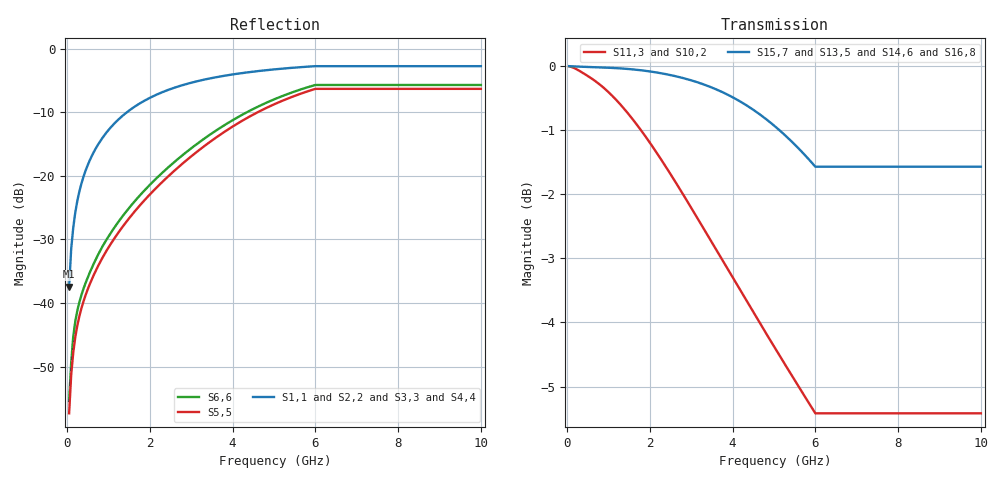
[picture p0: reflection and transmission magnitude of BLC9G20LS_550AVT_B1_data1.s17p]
! Created Mon Aug  3 12:37:55 2015
! 17 Port Network Data from SP1.SP block
! freq  magS1_1  angS1_1  magS1_2  angS1_2  magS1_3  angS1_3  magS1_4  angS1_4
!  magS1_5  angS1_5  magS1_6  angS1_6  magS1_7  angS1_7  magS1_8  angS1_8
!  magS1_9  angS1_9  magS1_10  angS1_10  magS1_11  angS1_11  magS1_12  angS1_12
!  magS1_13  angS1_13  magS1_14  angS1_14  magS1_15  angS1_15  magS1_16  angS1_16
!  magS1_17  angS1_17
!  magS2_1  angS2_1  magS2_2  angS2_2  magS2_3  angS2_3
!  magS2_4  angS2_4  magS2_5  angS2_5  magS2_6  angS2_6  magS2_7  angS2_7
!  magS2_8  angS2_8  magS2_9  angS2_9  magS2_10  angS2_10  magS2_11  angS2_11
!  magS2_12  angS2_12  magS2_13  angS2_13  magS2_14  angS2_14  magS2_15  angS2_15
!  magS2_16  angS2_16  magS2_17  angS2_17
!  magS3_1  angS3_1  magS3_2  angS3_2
!  magS3_3  angS3_3  magS3_4  angS3_4  magS3_5  angS3_5  magS3_6  angS3_6
!  magS3_7  angS3_7  magS3_8  angS3_8  magS3_9  angS3_9  magS3_10  angS3_10
!  magS3_11  angS3_11  magS3_12  angS3_12  magS3_13  angS3_13  magS3_14  angS3_14
!  magS3_15  angS3_15  magS3_16  angS3_16  magS3_17  angS3_17
!  magS4_1  angS4_1
!  magS4_2  angS4_2  magS4_3  angS4_3  magS4_4  angS4_4  magS4_5  angS4_5
!  magS4_6  angS4_6  magS4_7  angS4_7  magS4_8  angS4_8  magS4_9  angS4_9
!  magS4_10  angS4_10  magS4_11  angS4_11  magS4_12  angS4_12  magS4_13  angS4_13
!  magS4_14  angS4_14  magS4_15  angS4_15  magS4_16  angS4_16  magS4_17  angS4_17
!  magS5_1  angS5_1  magS5_2  angS5_2  magS5_3  angS5_3  magS5_4  angS5_4
!  magS5_5  angS5_5  magS5_6  angS5_6  magS5_7  angS5_7  magS5_8  angS5_8
!  magS5_9  angS5_9  magS5_10  angS5_10  magS5_11  angS5_11  magS5_12  angS5_12
!  magS5_13  angS5_13  magS5_14  angS5_14  magS5_15  angS5_15  magS5_16  angS5_16
!  magS5_17  angS5_17
!  magS6_1  angS6_1  magS6_2  angS6_2  magS6_3  angS6_3
!  magS6_4  angS6_4  magS6_5  angS6_5  magS6_6  angS6_6  magS6_7  angS6_7
!  magS6_8  angS6_8  magS6_9  angS6_9  magS6_10  angS6_10  magS6_11  angS6_11
!  magS6_12  angS6_12  magS6_13  angS6_13  magS6_14  angS6_14  magS6_15  angS6_15
!  magS6_16  angS6_16  magS6_17  angS6_17
!  magS7_1  angS7_1  magS7_2  angS7_2
!  magS7_3  angS7_3  magS7_4  angS7_4  magS7_5  angS7_5  magS7_6  angS7_6
!  magS7_7  angS7_7  magS7_8  angS7_8  magS7_9  angS7_9  magS7_10  angS7_10
!  magS7_11  angS7_11  magS7_12  angS7_12  magS7_13  angS7_13  magS7_14  angS7_14
!  magS7_15  angS7_15  magS7_16  angS7_16  magS7_17  angS7_17
!  magS8_1  angS8_1
!  magS8_2  angS8_2  magS8_3  angS8_3  magS8_4  angS8_4  magS8_5  angS8_5
!  magS8_6  angS8_6  magS8_7  angS8_7  magS8_8  angS8_8  magS8_9  angS8_9
!  magS8_10  angS8_10  magS8_11  angS8_11  magS8_12  angS8_12  magS8_13  angS8_13
!  magS8_14  angS8_14  magS8_15  angS8_15  magS8_16  angS8_16  magS8_17  angS8_17
!  magS9_1  angS9_1  magS9_2  angS9_2  magS9_3  angS9_3  magS9_4  angS9_4
!  magS9_5  angS9_5  magS9_6  angS9_6  magS9_7  angS9_7  magS9_8  angS9_8
!  magS9_9  angS9_9  magS9_10  angS9_10  magS9_11  angS9_11  magS9_12  angS9_12
!  magS9_13  angS9_13  magS9_14  angS9_14  magS9_15  angS9_15  magS9_16  angS9_16
!  magS9_17  angS9_17
!  magS10_1  angS10_1  magS10_2  angS10_2  magS10_3  angS10_3
!  magS10_4  angS10_4  magS10_5  angS10_5  magS10_6  angS10_6  magS10_7  angS10_7
!  magS10_8  angS10_8  magS10_9  angS10_9  magS10_10  angS10_10  magS10_11  angS10_11
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# ghz S ma R 50
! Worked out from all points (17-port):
!   200 points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, 50 MHz to 10 GHz, reference 50 ohm
!   strongest paths, dB at 50 MHz, 2.55 GHz, 5.05 GHz, 7.55 GHz, 10 GHz:
!     S15,7: 0.0, -0.1, -1.0, -1.6, -1.6
!     S13,5: 0.0, -0.1, -1.0, -1.6, -1.6
!     S14,6: 0.0, -0.2, -1.2, -1.8, -1.8
!     S16,8: 0.0, -0.2, -1.2, -1.8, -1.8
!     S11,3: 0.0, -1.7, -4.4, -5.4, -5.4
!     S10,2: 0.0, -1.7, -4.4, -5.4, -5.4
!   lowest |S11| = -37.4 dB at 50 MHz (marker M1), VSWR 1.03, Z = 49.9 - j1.34 ohm
!   |S11| at or under -10 dB: start of sweep to 1.442 GHz
